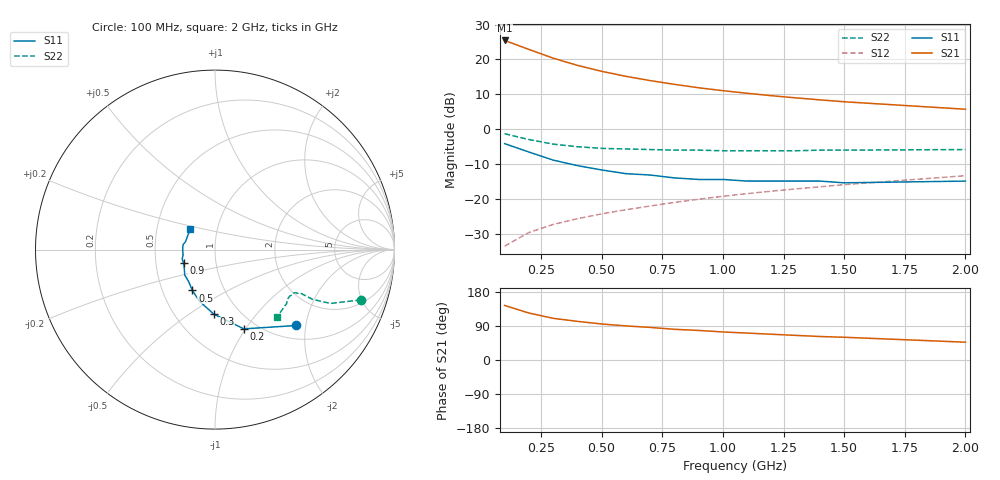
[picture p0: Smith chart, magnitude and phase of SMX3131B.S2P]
! HSMX-3131 Common Emitter
! Vce=10V Ic=10ma
# ghz s ma r 50
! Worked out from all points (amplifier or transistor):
!   16 points, 100 MHz to 2 GHz, reference 50 ohm
!   highest |S21| = 25.4 dB at 100 MHz (marker M1)
!   |S21| within 3 dB of that: start of sweep to 217.3 MHz
!   unconditionally stable (mu >= 1): 687.4 MHz to 1.845 GHz
!   at 300 MHz: K = 0.75, MSG = 23.8 dB, |S12| = -27.3 dB
!   at 900 MHz: K = 1.04, MAG = 14.8 dB, |S12| = -20.1 dB
!   at 2 GHz: K = 0.99, MSG = 9.5 dB, |S12| = -13.4 dB
!   lowest NFmin = 1.70 dB at 500 MHz
!   S11 on the Smith chart (normalised r, x): 100 MHz: 1.29, -1.77; 200 MHz: 0.87, -0.98; 300 MHz: 0.76, -0.63; 500 MHz: 0.71, -0.34; 900 MHz: 0.70, -0.11; 2 GHz: 0.74, +0.18
0.1  0.62 -43.0  18.69 144.0  0.021 71.0  0.86 -19.0
0.2  0.47 -70.0  13.91 124.0  0.033 65.0  0.71 -25.0
0.3  0.36 -91.0  10.42 110.0  0.043 64.0  0.61 -27.0
0.4  0.3 -107.0  8.22 102.0  0.052 66.0  0.56 -27.0
0.5  0.26 -119.0  6.75 95.0  0.061 67.0  0.53 -27.0
0.6  0.23 -130.0  5.72 90.0  0.07 68.0  0.52 -28.0
0.7  0.22 -140.0  4.97 86.0  0.079 69.0  0.51 -28.0
0.8  0.2 -149.0  4.39 81.0  0.089 70.0  0.5 -29.0
0.9  0.19 -157.0  3.92 78.0  0.099 70.0  0.5 -30.0
1  0.19 -164.0  3.56 74.0  0.109 71.0  0.49 -32.0
1.1  0.18 -171.0  3.27 71.0  0.119 71.0  0.49 -33.0
1.2  0.18 -178.0  3.02 68.0  0.129 71.0  0.49 -34.0
1.3  0.18 177.0  2.81 65.0  0.139 71.0  0.49 -35.0
1.4  0.18 171.0  2.63 62.0  0.149 71.0  0.5 -37.0
1.5  0.17 165.0  2.47 60.0  0.16 70.0  0.5 -39.0
2  0.18 140.0  1.93 47.0  0.215 68.0  0.51 -47.0
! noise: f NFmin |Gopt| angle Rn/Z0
0.5  1.7  0.36  -10  1.2
1  1.8  0.45  -130  0.04
1.5  2.1  0.32  31  0.14
2  3.3  0.5  -171  0.2
